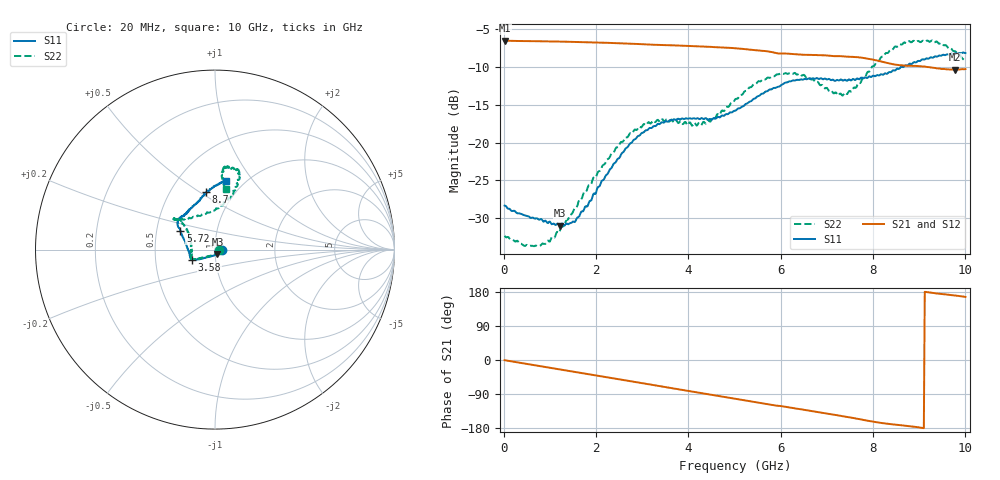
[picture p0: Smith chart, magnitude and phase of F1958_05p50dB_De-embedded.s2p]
! Integrated Device Technology
! Corporate Headquarters
! 6024 Silver Creek Valley Road
! San Jose, CA 95138  USA
! Phone:  1-408-284-8200
! Toll Free:  1-800-223-1366
! Webpage:  http://www.idt.com/
! Timing and RF Division
! 515 Groton Road, Suite 102
! Westford, MA 01886-6024
! Device:  F1958
! Description: 7-bit 0.25 dB Digital Step Attenuator
! Frequency:  0.001 -  6.000 GHz
! Package:  4x4 mm Thin QFN Plastic Package: 24 pin
! Ports:  2 RF, 12 DC
!  Pin  1  = D0
!  Pin  2  = VDD
!  Pin  3  = VMODE
!  Pin  4  = GND
!  Pin  5  = RF1  =  Port 1
!  Pin  6  = GND
!  Pin  7  = GND
!  Pin  8  = GND
!  Pin  9  = GND
!  Pin 10  = GND
!  Pin 11  = GND
!  Pin 12  = GND
!  Pin 13  = GND
!  Pin 14  = RF2  =  Port 2
!  Pin 15  = GND
!  Pin 16  = LE
!  Pin 17  = CLK
!  Pin 18  = DATA
!  Pin 19  = D6
!  Pin 20  = D5
!  Pin 21  = D4
!  Pin 22  = D3
!  Pin 23  = D2
!  Pin 24  = D1
! State:  22
! Atten State:  5.50 dB
! Voltage:  +3.30 Volts
! Current:  0.258 mA
! Data:  The device was measured on a F1958 evaluation board which has
!  individual transmission lines to the RF pins.  Data was collected
!  using a calibrated network analyzer.  The evaluation board was
!  de-embedded using Automatic Fixture Removal (AFR).
!  The reference plane is the edge of the package pin.
! Misc:
!  Action Tracker AT0419
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# GHz S dB R 50
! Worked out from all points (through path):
!   500 points, 20 MHz to 10 GHz, reference 50 ohm
!   highest |S21| = -6.57 dB at 20 MHz (marker M1); lowest = -10.4 dB at 9.78 GHz (marker M2)
!   group delay of S21, straight-line fit = 54.9 ps
!   lowest |S11| = -31.0 dB at 1.22 GHz (marker M3), VSWR 1.06, Z = 51.3 - j2.55 ohm
!   |S11| at or under -10 dB: start of sweep to 8.618 GHz; 8.622 GHz to 8.669 GHz (46.61 MHz wide, 0.539 % of centre)
!   |S22| runs from -33.7 to -6.5 dB; largest |S21 - S12| = 0.0012
!   S11 on the Smith chart (normalised r, x): 20 MHz: 1.08, -0.00; 3.58 GHz: 0.77, -0.09; 5.72 GHz: 0.66, +0.15; 8.7 GHz: 0.74, +0.53; 10 GHz: 0.82, +0.74
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0.02  -28.31 -3.1  -6.57 -0.6  -6.57 -0.5  -32.29 -4.7
0.76  -30.16 -27.8  -6.65 -15.6  -6.65 -15.6  -33.57 -49.3
1.22  -30.95 -61.0  -6.69 -25.0  -6.69 -25.0  -31.58 -94.4
1.52  -30.43 -88.7  -6.74 -31.1  -6.73 -31.1  -28.86 -117.7
1.7  -29.07 -103.1  -6.76 -34.7  -6.76 -34.7  -27.27 -127.9
2.6  -21.20 -144.8  -6.94 -53.0  -6.93 -53.0  -19.72 -151.8
2.94  -19.09 -150.3  -7.02 -60.0  -7.01 -60.0  -17.88 -153.9
3.36  -17.57 -154.2  -7.14 -68.4  -7.14 -68.5  -17.15 -157.1
3.58  -17.14 -156.6  -7.18 -72.8  -7.18 -72.9  -17.25 -161.2
4.32  -16.89 -167.0  -7.33 -87.8  -7.35 -87.9  -17.29 171.4
5.02  -15.80 170.4  -7.57 -102.2  -7.59 -102.2  -14.27 145.0
5.72  -13.20 151.5  -7.99 -116.6  -8.00 -116.6  -11.43 140.8
6.28  -11.81 144.8  -8.35 -127.0  -8.36 -127.0  -10.88 142.8
6.68  -11.55 139.7  -8.46 -134.6  -8.48 -134.5  -11.67 139.2
7.2  -11.80 132.3  -8.62 -145.2  -8.63 -145.1  -13.42 116.7
7.4  -11.73 129.5  -8.67 -149.5  -8.67 -149.4  -13.45 101.9
7.92  -11.27 117.3  -8.98 -161.0  -8.98 -161.0  -10.65 75.5
8.34  -10.73 107.0  -9.56 -168.7  -9.57 -168.8  -8.07 70.6
8.7  -9.82 99.0  -9.87 -173.3  -9.87 -173.2  -6.85 74.2
9.3  -8.81 86.9  -10.14 176.7  -10.14 176.7  -6.65 83.3
9.78  -8.23 82.4  -10.40 170.1  -10.41 170.1  -7.96 83.6
10  -8.21 81.3  -10.32 166.4  -10.35 166.5  -9.30 80.0
